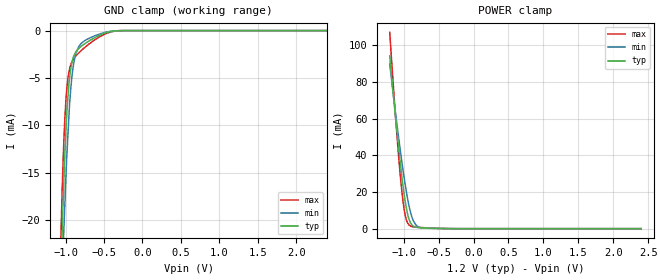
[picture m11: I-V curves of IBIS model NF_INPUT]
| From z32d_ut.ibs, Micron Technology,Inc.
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| MODEL NF_INPUT (Non-Functioning Terminator Model)
[Model]   NF_INPUT
Model_type   Terminator
|   typ   min   max
|C_comp   0.362pF   0.312pF   0.412pF
C_comp_power_clamp   0.181pF   0.156pF   0.206pF
C_comp_gnd_clamp   0.181pF   0.156pF   0.206pF
[Voltage Range]   1.2000V   1.1400V   1.2600V
| Junction Temperature (Ambient temp is 35C typ, 125C min, -40C max)
[Temperature Range]   50.0   140.0   -40.0
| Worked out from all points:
|   GND clamp passes 1 mA (typ) near -0.68 V on its own axis
|   POWER clamp passes 1 mA (typ) near -0.84 V on its own axis
[GND Clamp]
|   Voltage   I(typ)   I(min)   I(max)
-1.2V     -75.7mA    -73.15mA   -81.94mA
-1.06V    -25.47mA   -30.15mA   -21.29mA
-1.045V   -21.28mA   -26.41mA   -16.8mA
-1.025V   -16.24mA   -21.42mA   -12.02mA
-1.01V    -13.04mA   -18.29mA   -9.212mA
-980mV    -8.049mA   -12.51mA   -5.739mA
-950mV    -5.074mA   -7.962mA   -4.107mA
-920mV    -3.415mA   -5.011mA   -3.338mA
-865mV    -2.23mA    -2.372mA   -2.662mA
-775mV    -1.523mA   -1.197mA   -1.95mA
-315mV    -13.35uA   -11.28uA   -18.46uA
2.4V      0A         0A         0A
[POWER Clamp]
|   Voltage   I(typ)   I(min)   I(max)
-1.2V     94.24mA    89.76mA    107mA
-1.1V     54.19mA    57.92mA    52.68mA
-1.065V   41.3mA     47.43mA    35.99mA
-1.03V    29.43mA    37.45mA    21.62mA
-995mV    19.04mA    28.15mA    10.83mA
-975mV    14.08mA    23.29mA    6.744mA
-940mV    7.306mA    15.46mA    2.843mA
-910mV    3.836mA    10.08mA    1.58mA
-870mV    1.616mA    5.02mA     1.03mA
-830mV    856.5uA    2.219mA    837.6uA
-700mV    369.3uA    304.1uA    508.7uA
2.4V      0A         0A         0A
